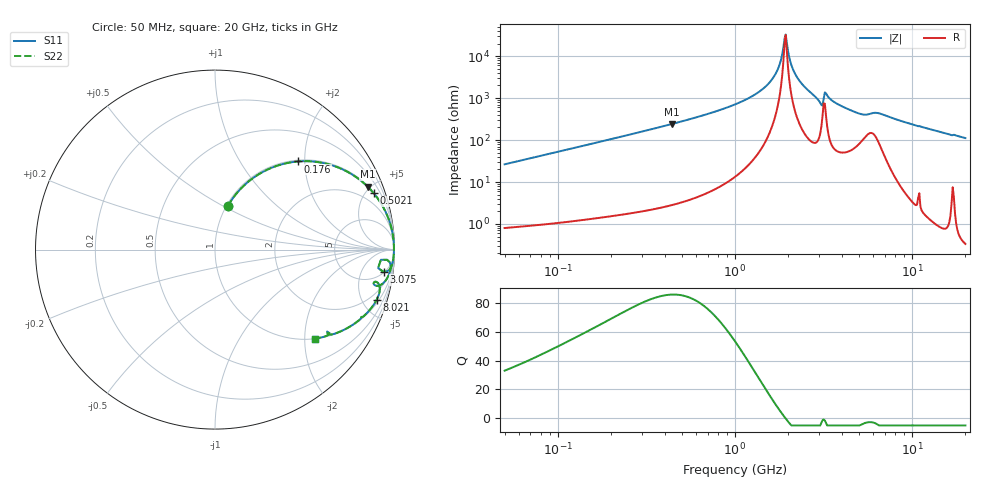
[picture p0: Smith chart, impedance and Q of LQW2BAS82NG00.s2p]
!Murata Part Number: LQW2BAS82NG00
!These Parameters are Measured in Series Mode Connection
!  o--[Z]--o
!Port1  Port2
!  o-------o
!Freq. Start=50[MHz] Stop=20[GHz], 401[Steps]
# Hz S RI R 50
!Freq.(Hz) S11(Real) S11(Imag) S21(Real) S21(Imag) S12(Real) S12(Imag) S22(Real) S22(Imag)
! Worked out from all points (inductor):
!   401 points, 50 MHz to 20 GHz, reference 50 ohm
!   read as one part in series: L = 83.8 nH near 51.52 MHz
!   highest Q = 85.7 at 438.7 MHz (marker M1), where L = 87.3 nH
!   self-resonance near 1.904 GHz
!   S11 on the Smith chart (normalised r, x): 50 MHz: 1.02, +0.53; 176 MHz: 1.03, +1.85; 502.1 MHz: 1.07, +5.60; 3.075 GHz: 5, -13; 8.021 GHz: 1.26, -6.34; 20 GHz: 1.01, -2.24
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5e7  0.0716 0.2432  0.9284 -0.2432  0.9284 -0.2432  0.0716 0.2432
1.364002e8  0.3425 0.466  0.6575 -0.466  0.6575 -0.466  0.3425 0.466
1.759554e8  0.4629 0.491  0.5371 -0.491  0.5371 -0.491  0.4629 0.491
3.721004e8  0.799 0.3949  0.201 -0.3949  0.201 -0.3949  0.799 0.3949
4.387496e8  0.8498 0.3514  0.1502 -0.3514  0.1502 -0.3514  0.8498 0.3514
5.020686e8  0.884 0.3145  0.116 -0.3145  0.116 -0.3145  0.884 0.3145
1e9  0.9779 0.1379  0.0221 -0.1379  0.0221 -0.1379  0.9779 0.1379
1.329223e9  0.9916 0.0759  0.00837 -0.0759  0.00837 -0.0759  0.9916 0.0759
1.590961e9  0.9958 0.0389  0.00418 -0.0389  0.00418 -0.0389  0.9958 0.0389
1.740566e9  0.9968 0.0207  0.0032 -0.0207  0.0032 -0.0207  0.9968 0.0207
1.875929e9  0.9971 0.00547  0.00293 -0.00547  0.00293 -0.00547  0.9971 0.00547
1.932977e9  0.997 -0.000635  0.00297 0.000635  0.00297 0.000635  0.997 -0.000635
2.083303e9  0.9966 -0.0161  0.00343 0.0161  0.00343 0.0161  0.9966 -0.0161
2.179053e9  0.996 -0.0255  0.00399 0.0255  0.00399 0.0255  0.996 -0.0255
2.728004e9  0.9882 -0.0779  0.0118 0.0779  0.0118 0.0779  0.9882 -0.0779
3.075291e9  0.9405 -0.1248  0.0595 0.1248  0.0595 0.1248  0.9405 -0.1248
3.314454e9  0.9778 -0.0813  0.0222 0.0813  0.0222 0.0813  0.9778 -0.0813
3.680849e9  0.9747 -0.1238  0.0253 0.1238  0.0253 0.1238  0.9747 -0.1238
4.748272e9  0.9316 -0.1916  0.0684 0.1916  0.0684 0.1916  0.9316 -0.1916
7.442007e9  0.9125 -0.2517  0.0875 0.2517  0.0875 0.2517  0.9125 -0.2517
8.020766e9  0.9005 -0.2799  0.0995 0.2799  0.0995 0.2799  0.9005 -0.2799
2e10  0.5554 -0.4954  0.4446 0.4954  0.4446 0.4954  0.5554 -0.4954
